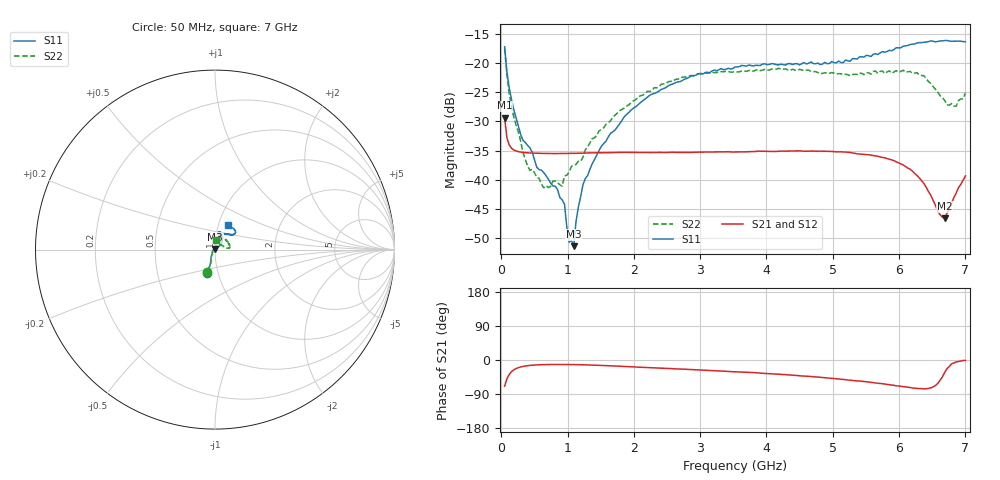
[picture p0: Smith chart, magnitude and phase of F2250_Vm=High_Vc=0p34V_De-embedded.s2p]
! Integrated Device Technology
! Corporate Headquarters
! 6024 Silver Creek Valley Road
! San Jose, CA 95138  USA
! Phone:  1-408-284-8200
! Toll Free:  1-800-223-1366
! Webpage:  http://www.idt.com/
! Timing and RF Division
! 515 Groton Road, Suite 102
! Westford, MA 01886-6024
! Device:  F2250
! Description: Voltage Variable RF Attenuator
! Frequency:  50.0 -  6000.00 MHz
! Package:  3x3 mm Thin QFN Plastic Package: 16 pin
! Ports:  2 RF, 3 DC
!  Pin  1  = GND
!  Pin  2  = NC
!  Pin  3  = RF1  = Port 1
!  Pin  4  = NC
!  Pin  5  = GND
!  Pin  6  = GND
!  Pin  7  = GND
!  Pin  8  = GND
!  Pin  9  = NC
!  Pin 10  = RF2  = Port 2
!  Pin 11  = NC
!  Pin 12  = GND
!  Pin 13  = GND
!  Pin 14  = VCNTRL
!  Pin 15  = VDD
!  Pin 16  = VMODE
! Vcntrl:  0.340 Volts
! Vmode:  +3.300 Volts
! Vdd:  +3.30  Volts
! Current:  1.259 mA
! Data:  The device was measured on a the F2250 evaluation board which has
!  individual transmission lines to the RF pins.  Data was collected
!  using a calibrated network analyzer.  The evaluation board was
!  de-embedded using a TRL calibration technique.
!  The reference plane is the edge of the package pin.
! Misc:  SN 10
!  Action Tracker AT0258
! Date Measured:  2014-11-26
! Date:  2015-10-15  MJV
! Note:
!  Integrated Device Technology supplies this data as a sample of measured
!  data at the package pin for this product.  Your particular data for this
!  product may vary.
!  Data was taken at 25 degrees C.
!  Integrated Device Technology reserves the right to change this data at anytime.
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# GHz S dB R 50
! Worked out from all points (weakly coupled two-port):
!   201 points, 50 MHz to 7 GHz, reference 50 ohm
!   highest |S21| = -29.35 dB at 50 MHz (marker M1); lowest = -46.6 dB at 6.687 GHz (marker M2)
!   lowest |S11| = -51.4 dB at 1.093 GHz (marker M3), VSWR 1.01, Z = 50 + j0.27 ohm
!   |S11| at or under -10 dB: start of sweep to end of sweep
!   |S22| runs from -41.4 to -17.5 dB; largest |S21 - S12| = 5.1e-05
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0.05  -17.18 -108.5  -29.35 -69.1  -29.35 -69.1  -17.51 -109.9
0.08475  -21.47 -107.4  -32.79 -49.7  -32.79 -49.7  -22.06 -107.5
0.189  -28.00 -119.9  -34.89 -26.0  -34.89 -26.0  -29.24 -120.8
0.328  -33.23 -134.1  -35.31 -16.9  -35.31 -16.9  -35.37 -135.5
0.43225  -34.54 -145.3  -35.40 -14.3  -35.40 -14.3  -38.37 -163.5
0.5365  -37.88 -154.7  -35.45 -12.9  -35.45 -12.9  -39.61 -178.2
0.64075  -38.77 -162.6  -35.48 -12.2  -35.47 -12.2  -41.39 157.0
0.91875  -43.44 155.8  -35.50 -11.8  -35.50 -11.8  -41.10 116.4
0.9535  -44.22 170.8  -35.50 -11.8  -35.50 -11.9  -39.32 114.0
1.023  -50.72 140.1  -35.49 -12.0  -35.49 -12.0  -38.69 96.2
1.0925  -51.39 89.4  -35.47 -12.1  -35.48 -12.1  -37.48 87.4
1.12725  -47.17 61.6  -35.47 -12.2  -35.46 -12.2  -37.36 80.3
1.2315  -40.86 40.6  -35.43 -12.6  -35.43 -12.6  -36.15 66.7
1.6485  -32.03 41.1  -35.34 -15.3  -35.34 -15.3  -29.87 54.9
2.37825  -24.75 46.7  -35.31 -21.2  -35.31 -21.2  -24.06 51.3
3.525  -20.66 71.7  -35.22 -30.9  -35.23 -30.9  -21.47 71.6
4.7065  -20.06 72.0  -35.07 -44.2  -35.08 -44.2  -21.46 69.6
5.85325  -17.79 40.5  -36.49 -65.2  -36.49 -65.2  -21.31 22.1
6.3745  -16.40 40.9  -40.63 -76.1  -40.65 -76.1  -22.13 5.9
6.68725  -16.11 47.9  -46.60 -33.0  -46.57 -32.8  -26.37 27.4
6.861  -16.22 54.5  -42.29 -5.2  -42.25 -5.2  -27.38 57.7
7  -16.32 62.4  -39.35 -1.3  -39.32 -1.5  -25.08 84.7
